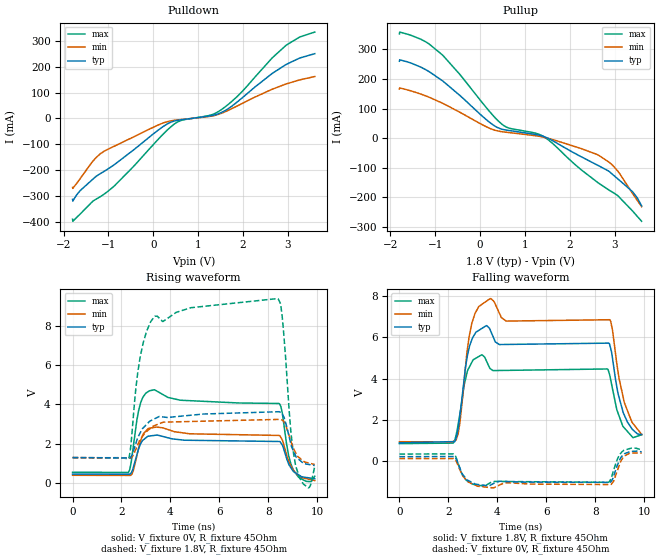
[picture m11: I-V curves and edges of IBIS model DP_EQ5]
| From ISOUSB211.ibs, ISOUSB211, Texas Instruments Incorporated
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[Model]   DP_EQ5
Model_type   Output
Polarity   Non-Inverting
Vmeas = 0.2
Vref = 0
Cref = 15pF
Rref = 45
|   typ   min   max
C_comp   5pF   3pF   8pF
[Voltage Range]   1.8   1.71   1.89
[Temperature Range]   27   150   -40
[Pullup Reference]   1.8   1.71   1.89
[Pulldown Reference]   0   0   0
[Power Clamp Reference]   1.8   1.71   1.89
[GND Clamp Reference]   0   0   0
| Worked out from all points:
|   slope of the pulldown table from 0 to 0.27 V, typ, clamps not added: 7.95 ohm
|   slope of the pullup table from 0 to 0.27 V, typ, clamps not added: 7.94 ohm
|   falling waveform, V_fixture 1.8V, R_fixture 45Ohm: 20-80 % time 72.6ps typ, 77.1ps min, 75.3ps max; typ from 0.895 V to 1.3 V
|   rising waveform, V_fixture 0V, R_fixture 45Ohm: 20-80 % time 393ps typ, 411ps min, 71.6ps max; typ from 0.46 V to 0.225 V
|   rising waveform, V_fixture 1.8V, R_fixture 45Ohm: 20-80 % time 292ps typ, 346ps min, 35.9ps max; typ from 1.3 V to 0.895 V
|   falling waveform, V_fixture 0V, R_fixture 45Ohm: 20-80 % time 183ps typ, 189ps min, 104ps max; typ from 0.225 V to 0.46 V
[Pulldown]
|   Voltage   I(typ)   I(min)   I(max)
-1.8V     -312.3mA   -266.2mA   -388.8mA
-1.795V   -319mA     -269.8mA   -396.8mA
-1.633V   -278.9mA   -232.8mA   -369.2mA
-1.179V   -212.7mA   -136mA     -301.6mA
-865.8mV  -177.8mA   -106.8mA   -260mA
73.8mV    -49.63mA   -27.98mA   -87.09mA
538.2mV   -7.266mA   -5.626mA   -13.71mA
1.294V    10.85mA    9.019mA    13.98mA
1.521V    23.18mA    20.15mA    34.45mA
1.899V    67.71mA    50.57mA    89.7mA
2.947V    206.8mA    132.3mA    280.4mA
3.6V      250.2mA    161.9mA    333.6mA
[Pullup]
|   Voltage   I(typ)   I(min)   I(max)
-1.8V     259.8mA    166.3mA    352.1mA
-1.795V   264.8mA    169.7mA    358.5mA
-1.325V   240.1mA    149.1mA    334.3mA
-849.6mV  194.9mA    118.9mA    282mA
381.6mV   36.3mA     24.84mA    61.51mA
613.8mV   26.64mA    19.55mA    35.63mA
1.402V    6.733mA    3.773mA    6.537mA
2.612V    -90.76mA   -55.24mA   -148.5mA
2.876V    -112.3mA   -81.28mA   -175.5mA
3.065V    -136.9mA   -110.7mA   -193.6mA
3.4V      -181.3mA   -187.3mA   -246.2mA
3.6V      -228.6mA   -231.2mA   -280.5mA
[Ramp]
R_load = 45
|   typ   min   max
dV/dt_r   0.140808/3.19248e-10   0.160407/3.2917e-10   0.120509/1.68237e-09
dV/dt_f   0.243789/6.82122e-11   0.210518/7.19651e-11   0.256824/7.33847e-09
[Falling Waveform]
V_fixture = 1.8V
V_fixture_min = 1.71V
V_fixture_max = 1.89V
R_fixture = 45Ohm
C_fixture = 0F
|   Time   V(typ)   V(min)   V(max)
0s        895mV      947.6mV    856.5mV
2.314ns   1.125V     1.03V      1.264V
2.653ns   4.054V     3.973V     3.727V
2.944ns   5.828V     6.592V     4.751V
3.382ns   6.43V      7.594V     5.144V
3.707ns   6.357V     7.862V     4.479V
4.367ns   5.647V     6.776V     4.394V
8.595ns   5.636V     6.842V     4.169V
9.186ns   2.248V     2.875V     1.622V
9.9ns     1.301V     1.298V     1.285V
[Rising Waveform]
V_fixture = 0V
V_fixture_min = 0V
V_fixture_max = 0V
R_fixture = 45Ohm
C_fixture = 0F
|   Time   V(typ)   V(min)   V(max)
0s        459.5mV    400.3mV    553.4mV
2.282ns   452.2mV    391.7mV    544.2mV
2.489ns   823.8mV    654.8mV    1.913V
2.774ns   1.975V     2.119V     4.044V
3.337ns   2.422V     2.829V     4.739V
4.388ns   2.205V     2.573V     4.213V
8.434ns   2.114V     2.421V     4.043V
9.027ns   590mV      657.1mV    665.8mV
9.547ns   290mV      231.1mV    92.71mV
9.9ns     224.9mV    133mV      352.5mV
[Rising Waveform]
V_fixture = 1.8V
V_fixture_min = 1.71V
V_fixture_max = 1.89V
R_fixture = 45Ohm
C_fixture = 0F
|   Time   V(typ)   V(min)   V(max)
0s        1.301V     1.298V     1.285V
2.289ns   1.279V     1.277V     1.229V
2.761ns   2.543V     2.197V     6.382V
3.348ns   3.265V     2.92V      8.462V
8.362ns   3.623V     3.233V     9.365V
8.562ns   3.533V     3.202V     8.534V
8.917ns   2.02V      2.153V     2.686V
9.111ns   1.404V     1.567V     942.7mV
9.63ns    953.5mV    1.031V     -237.6mV
9.9ns     895mV      947.6mV    856.5mV
[Falling Waveform]
|Gnd
V_fixture = 0V
V_fixture_min = 0V
V_fixture_max = 0V
R_fixture = 45Ohm
C_fixture = 0F
|   Time   V(typ)   V(min)   V(max)
0s        224.9mV    133mV      352.5mV
2.207ns   232.5mV    135.8mV    358.8mV
2.71ns    -816.5mV   -863.2mV   -886mV
3.454ns   -1.154V    -1.235V    -1.198V
3.895ns   -1.04V     -1.253V    -970.5mV
4.391ns   -973.2mV   -1.033V    -974.9mV
8.634ns   -994.4mV   -1.12V     -866.2mV
8.917ns   -155.9mV   -415.1mV   132.5mV
9.098ns   253.3mV    105.8mV    463.6mV
9.9ns     459.5mV    400.3mV    553.4mV
